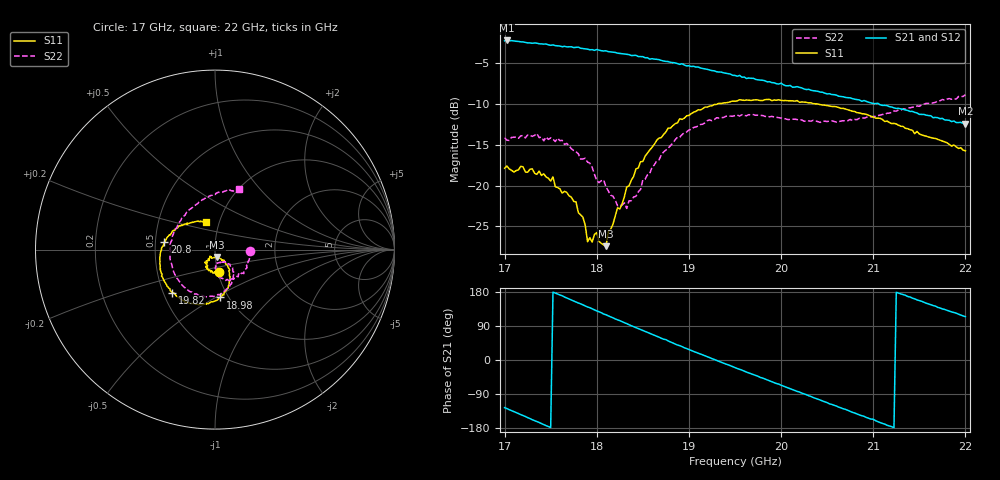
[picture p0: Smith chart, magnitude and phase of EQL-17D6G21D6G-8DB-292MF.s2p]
!Agilent Technologies,N5230C,MY49001174,A.09.42.21
!Agilent N5230C: A.09.42.21
!Date: Sunday, February 15, 2015 07:07:56
!Correction: S11(Full 2 Port(1,2))
!S21(Full 2 Port(1,2))
!S12(Full 2 Port(1,2))
!S22(Full 2 Port(1,2))
!S2P File: Measurements: S11, S21, S12, S22:
# Hz S  dB  R 50
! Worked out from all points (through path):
!   201 points, 17 GHz to 22 GHz, reference 50 ohm
!   highest |S21| = -2.18 dB at 17.02 GHz (marker M1); lowest = -12.4 dB at 22 GHz (marker M2)
!   lowest |S11| = -27.4 dB at 18.1 GHz (marker M3), VSWR 1.09, Z = 51 - j4.18 ohm
!   |S11| at or under -10 dB: start of sweep to 19.3 GHz; 20.41 GHz to end of sweep
!   |S22| runs from -22.8 to -8.8 dB; largest |S21 - S12| = 0.019
!   S11 on the Smith chart (normalised r, x): 17 GHz: 1.01, -0.26; 18.98 GHz: 0.92, -0.53; 19.82 GHz: 0.56, -0.30; 20.8 GHz: 0.56, +0.05; 22 GHz: 0.86, +0.28
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1.7e10  -17.85 -80.9  -2.23 -125.7  -2.20 -125.5  -14.12 -1.8
1.7025e10  -17.59 -83.5  -2.18 -128.2  -2.23 -128.7  -14.41 -4.8
1.7275e10  -17.99 -99.5  -2.49 -154.6  -2.42 -154.7  -13.81 -30.9
1.745e10  -18.92 -114.5  -2.61 -173.1  -2.67 -173.0  -14.02 -49.5
1.7625e10  -20.90 -120.5  -2.95 169.5  -2.83 168.2  -14.44 -66.0
1.7775e10  -21.99 -127.7  -3.03 153.0  -3.03 153.4  -15.82 -77.7
1.785e10  -23.87 -121.3  -3.17 145.5  -3.18 145.0  -16.72 -84.7
1.79e10  -26.86 -126.6  -3.25 139.9  -3.20 139.9  -17.11 -84.0
1.8e10  -25.73 -110.4  -3.29 129.5  -3.29 129.7  -19.35 -86.9
1.81e10  -27.42 -73.6  -3.45 119.3  -3.56 118.9  -20.17 -88.6
1.8125e10  -25.67 -64.8  -3.55 116.5  -3.53 116.3  -20.63 -87.1
1.8325e10  -20.14 -52.7  -3.88 96.1  -3.88 95.8  -22.79 -70.6
1.8675e10  -14.16 -65.3  -4.53 60.3  -4.58 59.7  -16.84 -47.0
1.8975e10  -11.43 -83.7  -5.30 30.2  -5.21 30.3  -13.40 -66.9
1.92e10  -10.36 -98.9  -5.72 8.6  -5.84 8.5  -12.01 -83.0
1.95e10  -9.64 -116.6  -6.47 -20.0  -6.45 -19.8  -11.39 -108.2
1.9825e10  -9.44 -134.7  -7.12 -50.1  -7.16 -50.3  -11.49 -136.6
2.035e10  -9.92 -163.1  -8.35 -99.2  -8.36 -99.1  -11.97 173.4
2.08e10  -10.90 171.7  -9.39 -140.1  -9.46 -140.3  -11.87 132.9
2.1175e10  -12.24 151.0  -10.30 -174.3  -10.33 -174.2  -11.09 107.2
2.1575e10  -13.92 131.8  -11.34 149.8  -11.35 149.9  -9.90 86.6
2.2e10  -15.72 108.3  -12.37 114.3  -12.38 114.5  -8.85 68.2
